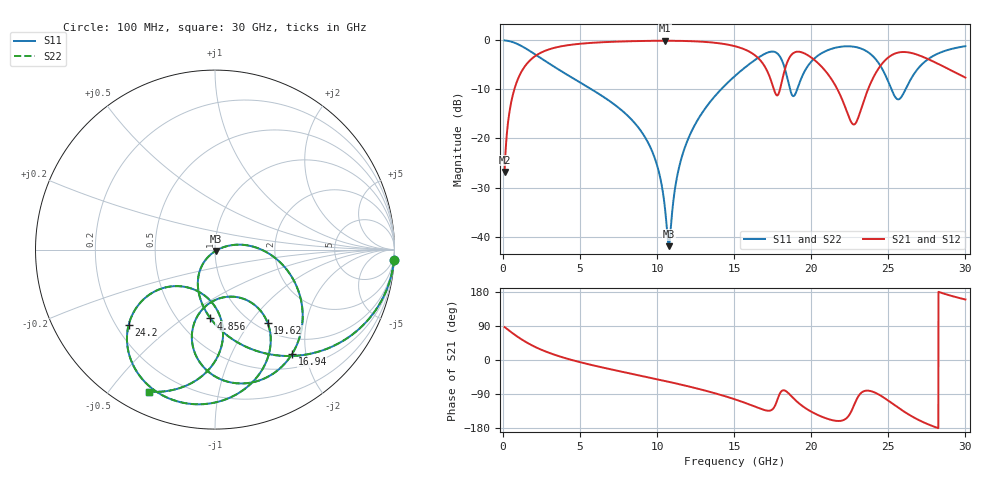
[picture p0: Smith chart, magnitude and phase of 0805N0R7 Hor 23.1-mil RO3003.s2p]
# GHz S MA R 50
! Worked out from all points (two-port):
!   3201 points, 100 MHz to 30 GHz, reference 50 ohm
!   highest |S21| = -0.07 dB at 10.5 GHz (marker M1); lowest = -26.8 dB at 100 MHz (marker M2)
!   |S21| within 3 dB of the highest: 2.141 GHz to 16.36 GHz (14.22 GHz wide, 154 % of centre); 25.18 GHz to 27.02 GHz (1.839 GHz wide, 7.05 % of centre)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
!   lowest |S11| = -42.0 dB at 10.75 GHz (marker M3), VSWR 1.02, Z = 50.4 - j0.7 ohm
!   |S11| at or under -10 dB: 5.753 GHz to 14.14 GHz (8.386 GHz wide, 84.3 % of centre); 18.63 GHz to 19.08 GHz (456.4 MHz wide, 2.42 % of centre); 25.21 GHz to 26.11 GHz (907.8 MHz wide, 3.54 % of centre)
!   |S22| runs from -42.0 to 0.0 dB; largest |S21 - S12| = 0
!   S11 on the Smith chart (normalised r, x): 100 MHz: 1, -36; 4.856 GHz: 0.71, -0.64; 16.94 GHz: 0.71, -1.75; 19.62 GHz: 1.13, -1.22; 24.2 GHz: 0.25, -0.35; 30 GHz: 0.09, -0.63
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0.1  0.9989 -3.2  0.04569 86.8  0.04569 86.8  0.9989 -3.2
0.5391563  0.9708 -16.9  0.2395 73.1  0.2395 73.1  0.9708 -16.9
1.296  0.8591 -38.0  0.5108 52.0  0.5108 52.0  0.8591 -38.0
4.855969  0.3841 -93.8  0.9197 -4.3  0.9197 -4.3  0.3841 -93.8
5.089563  0.3653 -96.1  0.9272 -6.7  0.9272 -6.7  0.3653 -96.1
10.06978  0.04827 -132.9  0.9914 -51.4  0.9914 -51.4  0.04827 -132.9
10.49959  0.01987 -122.7  0.9918 -55.3  0.9918 -55.3  0.01987 -122.7
10.75188  0.007984 -60.5  0.9917 -57.6  0.9917 -57.6  0.007984 -60.5
11.99459  0.09774 14.8  0.9847 -69.3  0.9847 -69.3  0.09774 14.8
15.05  0.4345 -17.6  0.8725 -103.9  0.8725 -103.9  0.4345 -17.6
16.93744  0.7237 -53.7  0.5563 -131.8  0.5563 -131.8  0.7237 -53.7
17.75969  0.7446 -83.4  0.2756 -109.5  0.2756 -109.5  0.7446 -83.4
18.27359  0.523 -104.2  0.4982 -80.5  0.4982 -80.5  0.523 -104.2
18.84356  0.2702 -78.7  0.744 -101.0  0.744 -101.0  0.2702 -78.7
19.61909  0.5009 -54.3  0.729 -127.0  0.729 -127.0  0.5009 -54.3
20.03956  0.6172 -60.0  0.6619 -137.3  0.6619 -137.3  0.6172 -60.0
22.73056  0.8638 -109.5  0.1391 -123.5  0.1391 -123.5  0.8638 -109.5
24.19753  0.6382 -138.9  0.469 -87.3  0.469 -87.3  0.6382 -138.9
25.01978  0.3719 -144.1  0.6746 -107.9  0.6746 -107.9  0.3719 -144.1
25.70188  0.2519 -110.6  0.7554 -127.4  0.7554 -127.4  0.2519 -110.6
26.80444  0.4882 -84.8  0.7215 -154.9  0.7215 -154.9  0.4882 -84.8
30  0.8736 -115.1  0.4178 159.7  0.4178 159.7  0.8736 -115.1
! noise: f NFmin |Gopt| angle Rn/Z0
0.1  0.001535  0.9658  1.477  0.01017
3.417  0.00769  0.7522  20.47  0.006066
6.743  0.01326  0.7248  37.76  0.008592
10.06  0.01981  0.7316  54.25  0.01173
13.39  0.03244  0.7826  69.96  0.02071
16.7  0.1203  0.9235  85.48  0.1881
20.03  0.1414  0.9238  100  0.1701
23.35  0.5597  0.9774  113.9  1.677
26.67  0.1727  0.9196  126.9  0.09543
30  0.1569  0.903  139.1  0.04411
